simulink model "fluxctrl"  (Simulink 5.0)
settings: Solver=ode45  StartTime=0.0  StopTime=0.04  MaxStep=1e-4  RelTol=1e-3
InitFcn:
  | close all,clear,clc,disp('Pre-loaded frequency and DC voltage'),fsw=50,Vdc=1,To=1/(6*fsw);
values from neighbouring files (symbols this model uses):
  To = 0.02    [fourier0.m]    (also in imdefSIvec1.m = 19.7882645911)
undefined symbols (not defined in the file or in its folder): Vdc
libraries: simulink x3

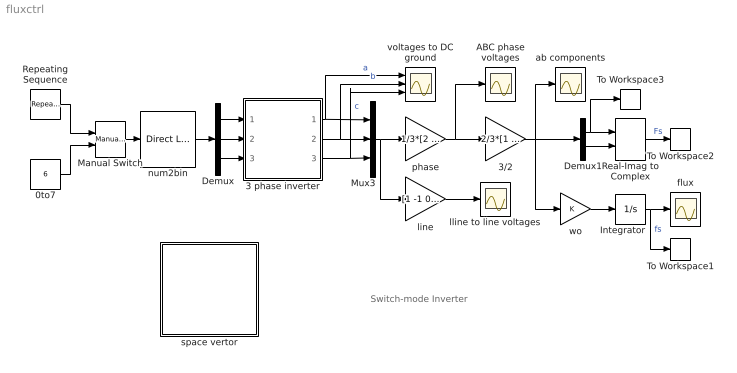
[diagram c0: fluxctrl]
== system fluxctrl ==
  note: Switch-mode Inverter
  0to7 : Constant  Value=6
  3 phase inverter : Subsystem
  3/2 : Gain  Gain=2/3*[1 -0.5 -0.5;0 sqrt(3)/2 -sqrt(3)/2]  Multiplication=Matrix(K*u)
  ABC phase voltages : Scope
  Demux : Demux  Outputs=3
  Demux1 : Demux  Outputs=2
  Integrator : Integrator  InitialCondition=[0 0]
  Manual Switch : simulink/Signal Routing/Manual Switch  sw=0  action=0
  Mux3 : Mux  Inputs=3
  Real-Imag to Complex : RealImagToComplex
  Repeating Sequence : simulink/Sources/Repeating Sequence  rep_seq_t="[0 1*To 1*To 2*To  2*To  3*To 3*To 4*To 4*To 5*To 5*To 6*To]"  rep_seq_y="[0 0 1 1 2  2 3  3 4 4 5 5]"
  To Workspace1 : ToWorkspace  VariableName=fs  SampleTime=-1  SaveFormat=Array
  To Workspace2 : ToWorkspace  VariableName=vs  SampleTime=-1  SaveFormat=Array
  To Workspace3 : ToWorkspace  VariableName=f  SampleTime=-1  SaveFormat=Array
  ab components : Scope
  flux : Scope
  line : Gain  Gain=[1 -1 0;0 1 -1;-1 0 1]  Multiplication=Matrix(K*u)
  lline to line voltages : Scope
  num2bin : simulink/Look-Up Tables/Direct Look-Up Table (n-D)  maskTabDims=2  explicitNumDims=1  outDims=Column  tabIsInput=off  mxTable=[1 0 1;1 0 0;1 1 0;0 1 0;0 1 1;0 0 1;0 0 0;1 1 1]'  clipFlag=Error
  phase : Gain  Gain=1/3*[2 -1 -1;-1 2 -1;-1 -1 2]  Multiplication=Matrix(K*u)
  space vertor : Subsystem
  voltages to DC ground : Scope  NumInputPorts=3
  wo : Gain
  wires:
  3/2/1 -> Demux1/1, ab components/1, wo/1
  Demux1/2 -> Real-Imag to Complex/2
  Demux1/1 -> Real-Imag to Complex/1, To Workspace3/1
  3 phase inverter/2(vb) -> Mux3/2, voltages to DC ground/2  "b"
  3 phase inverter/1(va) -> Mux3/1, voltages to DC ground/1  "a"
  3 phase inverter/3(vc) -> Mux3/3, voltages to DC ground/3  "c"
  Mux3/1 -> phase/1, line/1
  Real-Imag to Complex/1 -> To Workspace2/1  "Fs"
  num2bin/1 -> Demux/1
  Demux/1 -> 3 phase inverter/1(sa)
  Demux/2 -> 3 phase inverter/2(sb)
  Demux/3 -> 3 phase inverter/3(sc)
  phase/1 -> 3/2/1, ABC phase voltages/1
  line/1 -> lline to line voltages/1
  Manual Switch/1 -> num2bin/1
  0to7/1 -> Manual Switch/2
  Repeating Sequence/1 -> Manual Switch/1
  wo/1 -> Integrator/1
  Integrator/1 -> flux/1, To Workspace1/1  "fs"

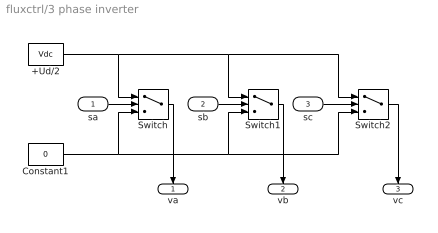
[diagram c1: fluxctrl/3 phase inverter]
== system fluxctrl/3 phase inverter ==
  sa : Inport
  sb : Inport  Port=2
  sc : Inport  Port=3
  +Ud/2 : Constant  Value=Vdc
  Constant1 : Constant  Value=0
  Switch : Switch  Threshold=0.5
  Switch1 : Switch  Threshold=0.5
  Switch2 : Switch  Threshold=0.5
  va : Outport  Orientation=down  InitialOutput=0
  vb : Outport  Orientation=down  Port=2  InitialOutput=0
  vc : Outport  Orientation=down  Port=3  InitialOutput=0
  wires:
  Switch1/1 -> vb/1
  Switch2/1 -> vc/1
  sc/1 -> Switch2/2
  sb/1 -> Switch1/2
  Switch/1 -> va/1
  sa/1 -> Switch/2
  Constant1/1 -> Switch2/3, Switch1/3, Switch/3
  +Ud/2/1 -> Switch2/1, Switch1/1, Switch/1

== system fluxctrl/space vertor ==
